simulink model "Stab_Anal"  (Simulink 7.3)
settings: Solver=ode45  StartTime=0.0  StopTime=500  RelTol=1e-3
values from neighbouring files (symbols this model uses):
  Ave = [    [vehicle_sim.m]
  Bve = [    [vehicle_sim.m]
  calfa = cos(alfa0*d2r)    [init.m]
  Cve = [    [vehicle_sim.m]
  d2r = pi/180    (= 0.0174532925199)    [init.m]    (also in robust.m)
  Dve = [    [vehicle_sim.m]
  ge = 32.174    [init.m]
  salfa = sin(alfa0*d2r)    [init.m]
  Thet0 = 27.69    [init.m]
  V0 = 24675.1    [init.m]
undefined symbols (not defined in the file or in its folder): Kmix, Kpr, Kq

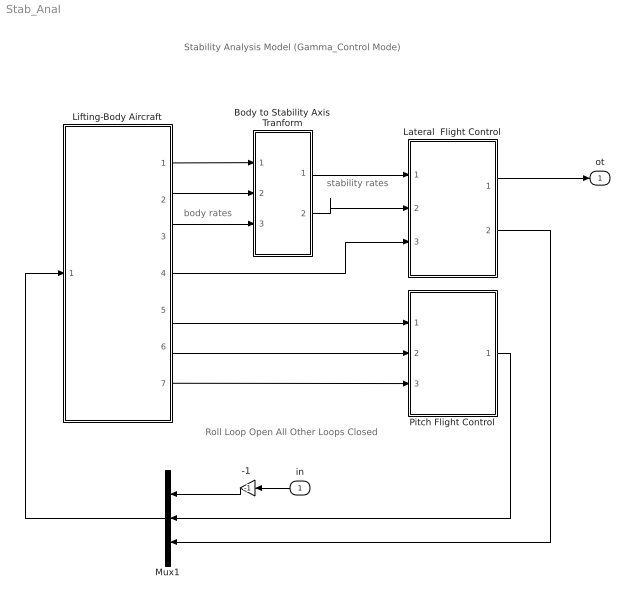
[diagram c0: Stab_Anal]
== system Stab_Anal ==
  note: Stability Analysis Model (Gamma_Control Mode)
  note: Roll Loop Open All Other Loops Closed
  note: body rates
  note: stability rates
  in : Inport  OutDataType=sfix(16)  OutScaling=2^0
  "-1 " : Gain  Gain=-1  ParameterDataType=sfix(16)  ParameterScaling=2^0  OutDataType=sfix(16)  OutScaling=2^0
  Body to Stability Axis Tranform : Subsystem
  Lateral  Flight Control : Subsystem
  Lifting-Body Aircraft : Subsystem
  Mux1 : Mux  Inputs=3
  Pitch Flight Control : Subsystem
  ot : Outport  OutDataType=sfix(16)  OutScaling=2^0
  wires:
  in/1 -> "-1 "/1
  Lifting-Body Aircraft/1(phi) -> Body to Stability Axis Tranform/1(phi)
  Lifting-Body Aircraft/3(r) -> Body to Stability Axis Tranform/3(r_b)
  Body to Stability Axis Tranform/2(r_s) -> Lateral  Flight Control/2(rs)
  Lifting-Body Aircraft/4(bet) -> Lateral  Flight Control/3(beta)
  Lifting-Body Aircraft/5(gam) -> Pitch Flight Control/1(gam)
  Lifting-Body Aircraft/6(q) -> Pitch Flight Control/2(q)
  Body to Stability Axis Tranform/1(p_s) -> Lateral  Flight Control/1(ps)
  Lifting-Body Aircraft/2(p) -> Body to Stability Axis Tranform/2(p_b)
  Lifting-Body Aircraft/7(Nz) -> Pitch Flight Control/3(Nz)
  Mux1/1 -> Lifting-Body Aircraft/1(PQR dem)
  Lateral  Flight Control/2(dR) -> Mux1/3
  Lateral  Flight Control/1(dP) -> ot/1
  "-1 "/1 -> Mux1/1
  Pitch Flight Control/1(dQ) -> Mux1/2

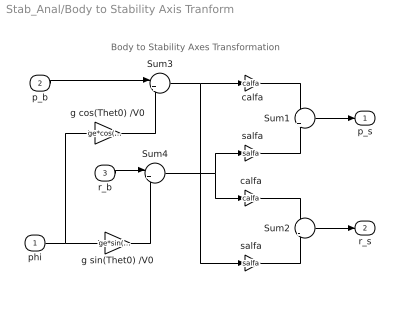
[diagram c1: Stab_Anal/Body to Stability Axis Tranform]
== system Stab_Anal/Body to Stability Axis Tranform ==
  note: Body to Stability Axes Transformation
  phi : Inport  OutDataType=sfix(16)  OutScaling=2^0
  p_b : Inport  Port=2  OutDataType=sfix(16)  OutScaling=2^0
  r_b : Inport  Port=3  OutDataType=sfix(16)  OutScaling=2^0
  Sum1 : Sum  Inputs=+|+  OutDataType=sfix(16)  OutScaling=2^0
  Sum2 : Sum  Inputs=+|-  OutDataType=sfix(16)  OutScaling=2^0
  Sum3 : Sum  Inputs=|++  OutDataType=sfix(16)  OutScaling=2^0
  Sum4 : Sum  Inputs=|+-  OutDataType=sfix(16)  OutScaling=2^0
  calfa : Gain  Gain=calfa  ParameterDataType=sfix(16)  ParameterScaling=2^0  OutDataType=sfix(16)  OutScaling=2^0
  "calfa " : Gain  Gain=calfa  ParameterDataType=sfix(16)  ParameterScaling=2^0  OutDataType=sfix(16)  OutScaling=2^0
  g cos(Thet0) /V0 : Gain  Gain=ge*cos(Thet0*d2r)/V0  ParameterDataType=sfix(16)  ParameterScaling=2^0  OutDataType=sfix(16)  OutScaling=2^0
  g sin(Thet0) /V0 : Gain  Gain=ge*sin(Thet0*d2r)/V0  ParameterDataType=sfix(16)  ParameterScaling=2^0  OutDataType=sfix(16)  OutScaling=2^0
  salfa : Gain  Gain=salfa  ParameterDataType=sfix(16)  ParameterScaling=2^0  OutDataType=sfix(16)  OutScaling=2^0
  "salfa " : Gain  Gain=salfa  ParameterDataType=sfix(16)  ParameterScaling=2^0  OutDataType=sfix(16)  OutScaling=2^0
  p_s : Outport  OutDataType=sfix(16)  OutScaling=2^0
  r_s : Outport  Port=2  OutDataType=sfix(16)  OutScaling=2^0
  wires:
  Sum1/1 -> p_s/1
  Sum2/1 -> r_s/1
  p_b/1 -> Sum3/1
  r_b/1 -> Sum4/1
  g cos(Thet0) /V0/1 -> Sum3/2
  g sin(Thet0) /V0/1 -> Sum4/2
  phi/1 -> g cos(Thet0) /V0/1, g sin(Thet0) /V0/1
  Sum4/1 -> "calfa "/1, salfa/1
  Sum3/1 -> "salfa "/1, calfa/1
  calfa/1 -> Sum1/1
  salfa/1 -> Sum1/2
  "calfa "/1 -> Sum2/1
  "salfa "/1 -> Sum2/2

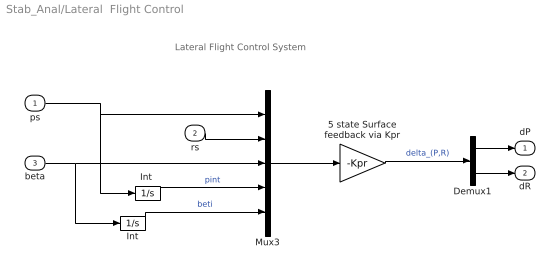
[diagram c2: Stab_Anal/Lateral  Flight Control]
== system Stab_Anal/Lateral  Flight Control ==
  note: Lateral Flight Control System
  ps : Inport  OutDataType=sfix(16)  OutScaling=2^0
  rs : Inport  Port=2  OutDataType=sfix(16)  OutScaling=2^0
  beta : Inport  Port=3  OutDataType=sfix(16)  OutScaling=2^0
  5 state Surface feedback via Kpr : Gain  Gain=-Kpr  Multiplication=Matrix(K*u)  ParameterDataType=sfix(16)  ParameterScaling=2^0  OutDataType=sfix(16)  OutScaling=2^0
  Demux1 : Demux  Outputs=2
  Int : Integrator
  "Int " : Integrator
  Mux3 : Mux  Inputs=5
  dP : Outport  OutDataType=sfix(16)  OutScaling=2^0
  dR : Outport  Port=2  OutDataType=sfix(16)  OutScaling=2^0
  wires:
  Demux1/2 -> dR/1
  Demux1/1 -> dP/1
  "Int "/1 -> Mux3/4  "pint"
  Int/1 -> Mux3/5  "beti"
  beta/1 -> Int/1, Mux3/3
  ps/1 -> "Int "/1, Mux3/1
  rs/1 -> Mux3/2
  5 state Surface feedback via Kpr/1 -> Demux1/1  "delta_(P,R)"
  Mux3/1 -> 5 state Surface feedback via Kpr/1

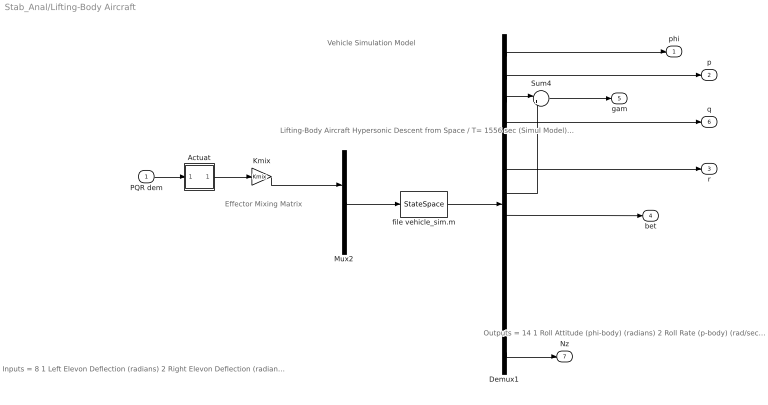
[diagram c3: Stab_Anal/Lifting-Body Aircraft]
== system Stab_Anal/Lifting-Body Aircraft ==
  note: Inputs = 8 1 Left Elevon Deflection (radians) 2 Right Elevon Deflection (radians) 3 Rudder Deflection (radians) 4 Upper Left Body-Flap Deflection (radians) 5 Upper Right Body-Flap Deflection (radians) 6 Lower Left Body-Flap Deflection (radians) 7 Lower Right Body-Flap Deflection (radians) 8 Wind Gust Azim, Elev Angles=(45 , 90) (deg)
  note: Lifting-Body Aircraft Hypersonic Descent from Space / T= 1556 sec (Simul Model) Gamma_Control Phase
  note: Effector Mixing Matrix
  note: Outputs = 14 1 Roll Attitude (phi-body) (radians) 2 Roll Rate (p-body) (rad/sec) 3 Pitch Attitude (thet-bdy) (radians) 4 Pitch Rate (q-body) (rad/sec) 5 Yaw Attitude (psi-body) (radians) 6 Yaw Rate (r-body) (rad/sec) 7 Angle of attack, alfa, (radians) 8 Angle of sideslip, beta, (radian) 9 Change in Altitude, delta-h, (feet) 10 Forward Acceleration (V-dot) (ft/sec) 11 Cross Range Velocity (Vcr) (ft/sec) 12 CG Acceleration along X axis, (ft/sec^2) 13 CG Acceleration along Y axis, (ft/sec^2) 14 CG Acceleration along Z axis, (ft/sec^2)
  note: Vehicle Simulation Model
  PQR dem : Inport  OutDataType=sfix(16)  OutScaling=2^0
  Actuat : Subsystem
  Demux1 : Demux  Outputs=14
  Kmix : Gain  Gain=Kmix  Multiplication=Matrix(K*u)  ParameterDataType=sfix(16)  ParameterScaling=2^0  OutDataType=sfix(16)  OutScaling=2^0
  Mux2 : Mux  Inputs=[7, 1]
  Sum4 : Sum  Inputs=|+-  OutDataType=sfix(16)  OutScaling=2^0
  file vehicle_sim.m : StateSpace  A=Ave  B=Bve  C=Cve  D=Dve
  phi : Outport  OutDataType=sfix(16)  OutScaling=2^0
  p : Outport  Port=2  OutDataType=sfix(16)  OutScaling=2^0
  r : Outport  Port=3  OutDataType=sfix(16)  OutScaling=2^0
  bet : Outport  Port=4  OutDataType=sfix(16)  OutScaling=2^0
  gam : Outport  Port=5  OutDataType=sfix(16)  OutScaling=2^0
  q : Outport  Port=6  OutDataType=sfix(16)  OutScaling=2^0
  Nz : Outport  Port=7  OutDataType=sfix(16)  OutScaling=2^0
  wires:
  Actuat/1(ou) -> Kmix/1
  Demux1/7 -> Sum4/2
  Sum4/1 -> gam/1
  Demux1/3 -> Sum4/1
  file vehicle_sim.m/1 -> Demux1/1
  Demux1/1 -> phi/1
  PQR dem/1 -> Actuat/1(in)
  Demux1/8 -> bet/1
  Demux1/6 -> r/1
  Demux1/4 -> q/1
  Demux1/2 -> p/1
  Kmix/1 -> Mux2/1
  Mux2/1 -> file vehicle_sim.m/1
  Demux1/14 -> Nz/1

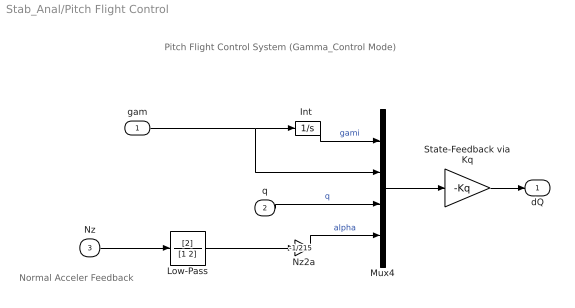
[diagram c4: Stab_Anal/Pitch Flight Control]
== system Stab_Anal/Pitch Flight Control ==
  note: Normal Acceler Feedback
  note: Pitch Flight Control System (Gamma_Control Mode)
  gam : Inport  OutDataType=sfix(16)  OutScaling=2^0
  q : Inport  Port=2  OutDataType=sfix(16)  OutScaling=2^0
  Nz : Inport  Port=3  OutDataType=sfix(16)  OutScaling=2^0
  " Nz2a" : Gain  Gain=-1/215  ParameterDataType=sfix(16)  ParameterScaling=2^0  OutDataType=sfix(16)  OutScaling=2^0
  "Int " : Integrator
  Low-Pass : TransferFcn  Numerator=[2]  Denominator=[1 2]
  Mux4 : Mux
  State-Feedback via Kq : Gain  Gain=-Kq  Multiplication=Matrix(K*u)  ParameterDataType=sfix(16)  ParameterScaling=2^0  OutDataType=sfix(16)  OutScaling=2^0
  dQ : Outport  OutDataType=sfix(16)  OutScaling=2^0
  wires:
  Low-Pass/1 -> " Nz2a"/1
  " Nz2a"/1 -> Mux4/4  "alpha"
  Nz/1 -> Low-Pass/1
  gam/1 -> Mux4/2, "Int "/1
  "Int "/1 -> Mux4/1  "gami"
  q/1 -> Mux4/3  "q"
  Mux4/1 -> State-Feedback via Kq/1
  State-Feedback via Kq/1 -> dQ/1

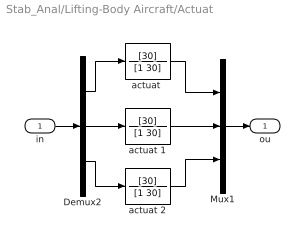
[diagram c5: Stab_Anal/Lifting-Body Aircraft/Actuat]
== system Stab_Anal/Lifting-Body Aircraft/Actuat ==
  in : Inport
  Demux2 : Demux  Outputs=3
  Mux1 : Mux  Inputs=3
  "actuat " : TransferFcn  Numerator=[30]  Denominator=[1 30]
  actuat 1 : TransferFcn  Numerator=[30]  Denominator=[1 30]
  actuat 2 : TransferFcn  Numerator=[30]  Denominator=[1 30]
  ou : Outport
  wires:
  Mux1/1 -> ou/1
  in/1 -> Demux2/1
  Demux2/3 -> actuat 2/1
  Demux2/1 -> "actuat "/1
  Demux2/2 -> actuat 1/1
  actuat 2/1 -> Mux1/3
  "actuat "/1 -> Mux1/1
  actuat 1/1 -> Mux1/2
